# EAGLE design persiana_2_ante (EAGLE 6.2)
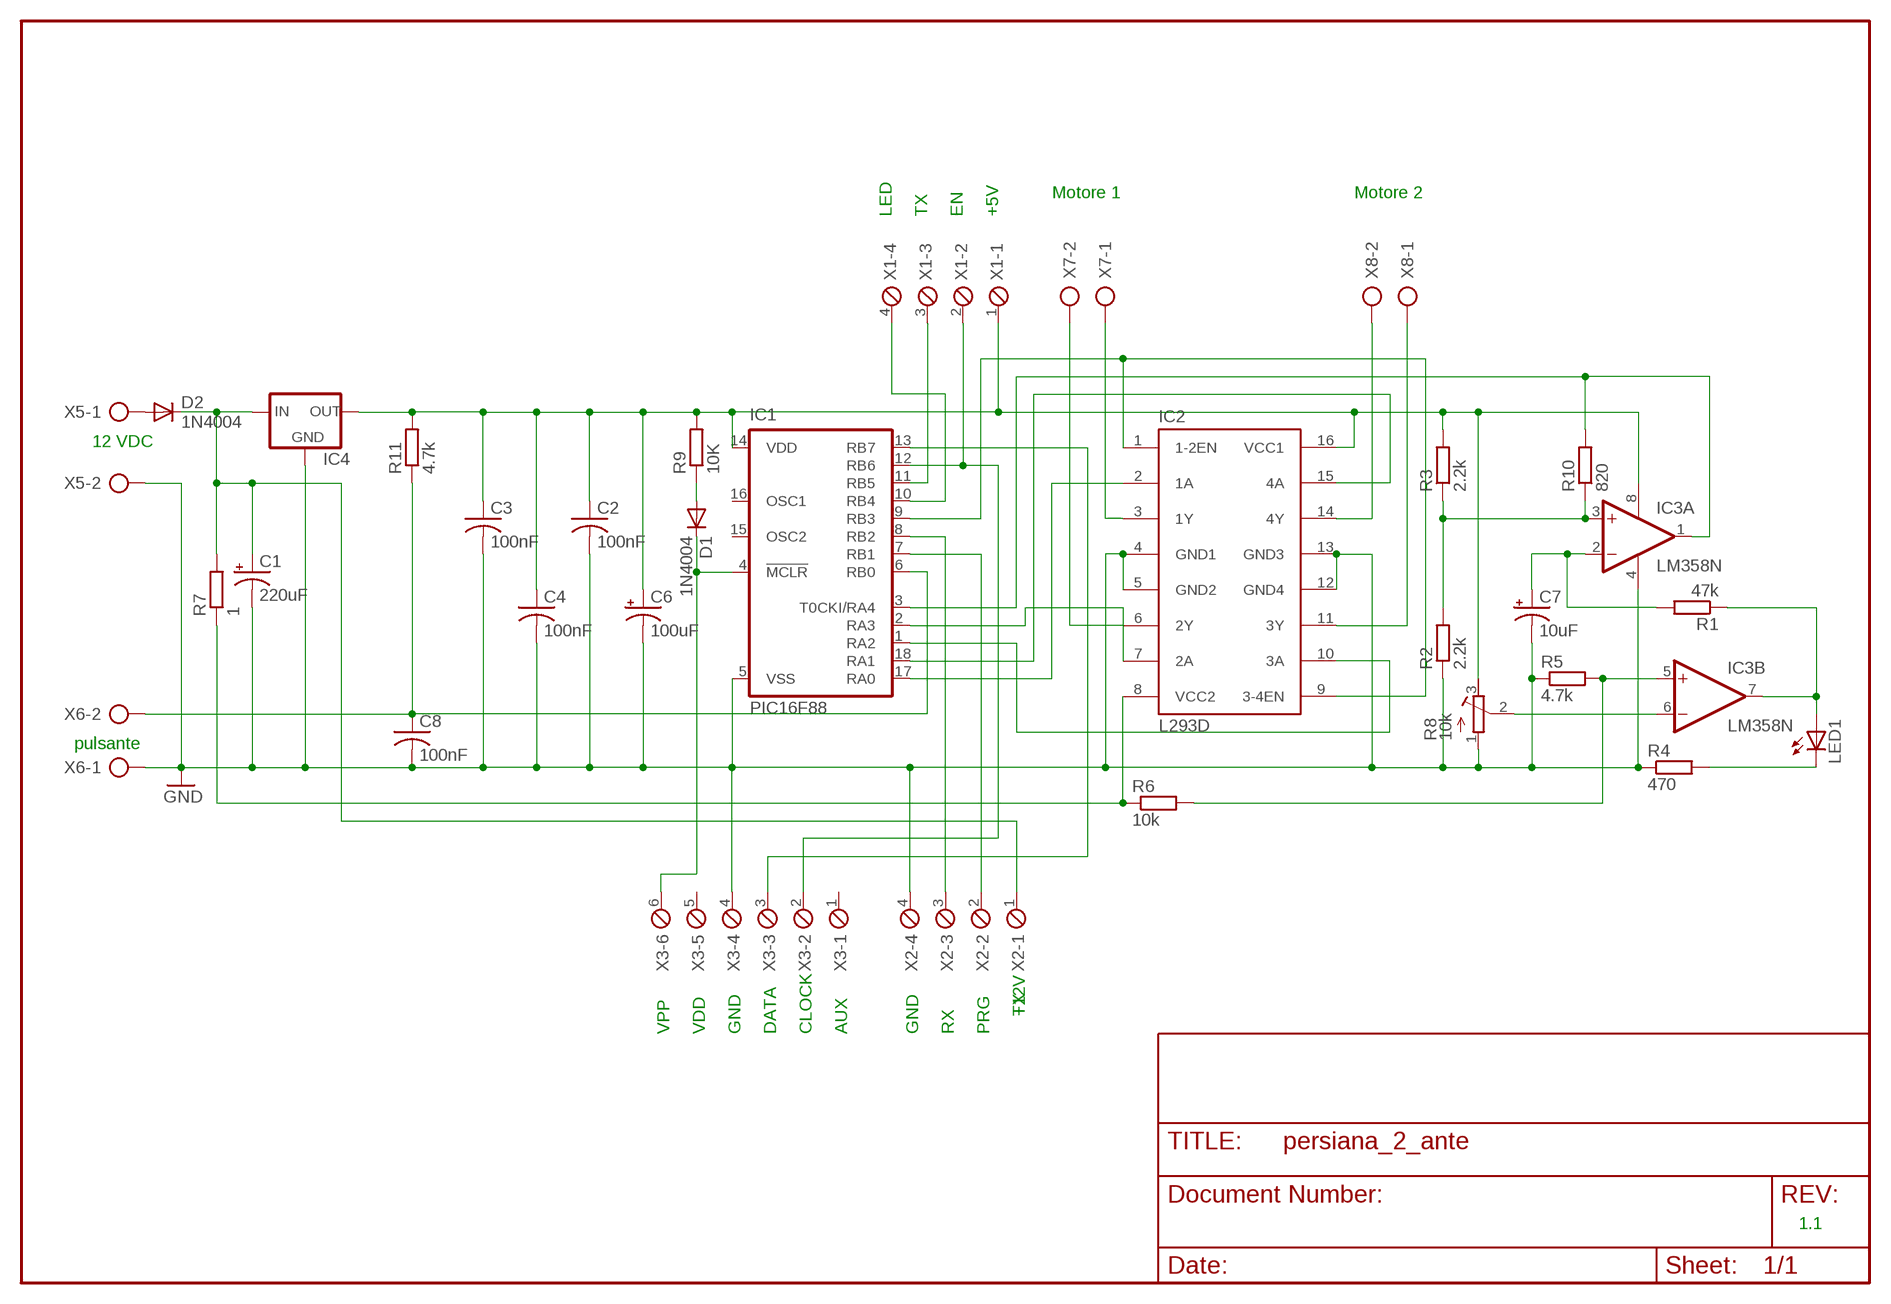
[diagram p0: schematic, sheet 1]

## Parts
C1  220uF  CPOL-USE5-10.5  [E5-10,5]
C2  100nF  C-US050-024X044  [C050-024X044]
C3  100nF  C-US050-024X044  [C050-024X044]
C4  100nF  C-US050-024X044  [C050-024X044]
C6  100uF  CPOL-USE5-10.5  [E5-10,5]
C7  10uF  CPOL-USE5-8.5  [E5-8,5]
C8  100nF  C-US050-024X044  [C050-024X044]
D1  1N4004  [DO41-10]
D2  1N4004  [DO41-10]
IC1  PIC16F88  PIC16F84AP  [DIL18]
IC2  L293D  [DIL16]
IC3  LM358N  [DIL08]
IC4  78XXS  [78XXS]
LED1  LED3MM  [LED3MM]
R1  47k  R-EU_0207/10  [0207/10]
R2  2.2k  R-EU_0207/10  [0207/10]
R3  2.2k  R-EU_0207/10  [0207/10]
R4  470  R-EU_0207/10  [0207/10]
R5  4.7k  R-EU_0207/10  [0207/10]
R6  10k  R-EU_0207/10  [0207/10]
R7  1  R-EU_0411/15  [0411/15]
R8  10k  R-TRIMM3296W  [RTRIM3296W]
R9  10K  R-EU_0207/10  [0207/10]
R10  820  R-EU_0207/10  [0207/10]
R11  4.7k  R-EU_0207/10  [0207/10]
X1  MPT4  [4POL254]
X2  MPT4  [4POL254]
X3  MPT6  [6POL254]
X5  AK500/2  [AK500/2]
X6  AK500/2  [AK500/2]
X7  AK500/2  [AK500/2]
X8  AK500/2  [AK500/2]

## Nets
GND: C1.- C2.2 C3.2 C4.2 C6.- C7.- C8.2 IC1.5(VSS) IC2.4(GND1) IC2.5(GND2) IC2.12(GND4) IC2.13(GND3) IC3.4(P:V-) IC4.GND R2.1 R4.1 R5.1 R8.1(E) X2.4 X3.4 X5.2 X6.1
N$1: C1.+ D2.C IC4.IN R7.2 X2.1
N$2: IC2.3(1Y) X7.1
N$3: IC2.6(2Y) X7.2
N$4: C8.1 IC1.6(RB0) R11.1 X6.2
N$6: D1.C IC1.4(!MCLR) X3.6
N$7: IC2.14(4Y) X8.2
N$8: C2.1 C3.1 C4.1 C6.+ IC1.14(VDD) IC2.16(VCC1) IC3.8(P:V+) IC4.OUT R3.2 R8.3(A) R9.2 R11.2 X1.1
N$9: IC2.8(VCC2) R6.1 R7.1
N$10: IC2.11(3Y) X8.1
N$11: IC1.13(RB7) X3.3
N$12: IC1.17(RA0) IC2.2(1A)
N$13: IC1.18(RA1) IC2.15(4A)
N$14: IC1.1(RA2) IC2.10(3A)
N$15: IC1.2(RA3) IC2.7(2A)
N$16: IC3.5(B:+IN) R5.2 R6.2
N$17: IC3.6(B:-IN) R8.2(S)
N$18: C7.+ IC3.2(A:-IN) R1.2
N$19: IC3.7(B:OUT) LED1.A R1.1
N$20: IC3.3(A:+IN) R2.2 R3.1 R10.1
N$21: IC1.11(RB5) X1.3
N$22: IC1.7(RB1) X2.2
N$23: IC1.3(T0CKI/RA4) IC3.1(A:OUT) R10.2
N$24: IC1.8(RB2) X2.3
N$25: LED1.K(C) R4.2
N$26: IC1.10(RB4) X1.4
N$27: D1.A R9.1
N$28: D2.A X5.1
N$42: IC1.9(RB3) IC2.1(1-2EN) IC2.9(3-4EN)
N$43: IC1.12(RB6) X1.2 X3.2
Unconnected: IC1.15(OSC2) IC1.16(OSC1) X3.1 X3.5

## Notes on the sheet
- Motore 1 | Motore 2
- LED | TX | EN | +5V
- 12 VDC
- pulsante
- +12V | TX
- VPP | VDD | GND | DATA | CLOCK | AUX | GND | RX | PRG
- 1.1

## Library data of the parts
C1 C6 C7 = rcl:CPOL-US: POLARIZED CAPACITOR, American symbol
C2-C4 C8 = rcl:C-US: CAPACITOR, American symbol
D1 D2 = diode:1N4004: DIODE
IC1 = microchip:PIC16F8*: MICROCONTROLLER 8-Bit PIC16F8X Family - CMOS Flash/EEPROM Pin Compatible : PIC16F83, PIC16CR83, PIC16F84A, PIC16CR84 see also PIC16C*
IC2 = st-microelectronics:L293D: PUSH-PULL 4 CHANNEL DRIVER
IC3 = linear:LM358: OP AMP
IC4 = v-reg:78XXS: VOLTAGE REGULATOR
LED1 = led:LED: LED
R1-R7 R9-R11 = rcl:R-EU_: RESISTOR, European symbol
R8 = rcl:R-TRIMM: Trimm resistor
X1 X2 = con-phoenix-254:MPT4: PHOENIX CONNECTOR; OC_FARNELL: unknown; OC_NEWARK: unknown
X3 = con-phoenix-254:MPT6: PHOENIX CONNECTOR; OC_FARNELL: unknown; OC_NEWARK: unknown
X5-X8 = con-ptr500:AK500/2: CONNECTOR; OC_FARNELL: unknown; OC_NEWARK: unknown

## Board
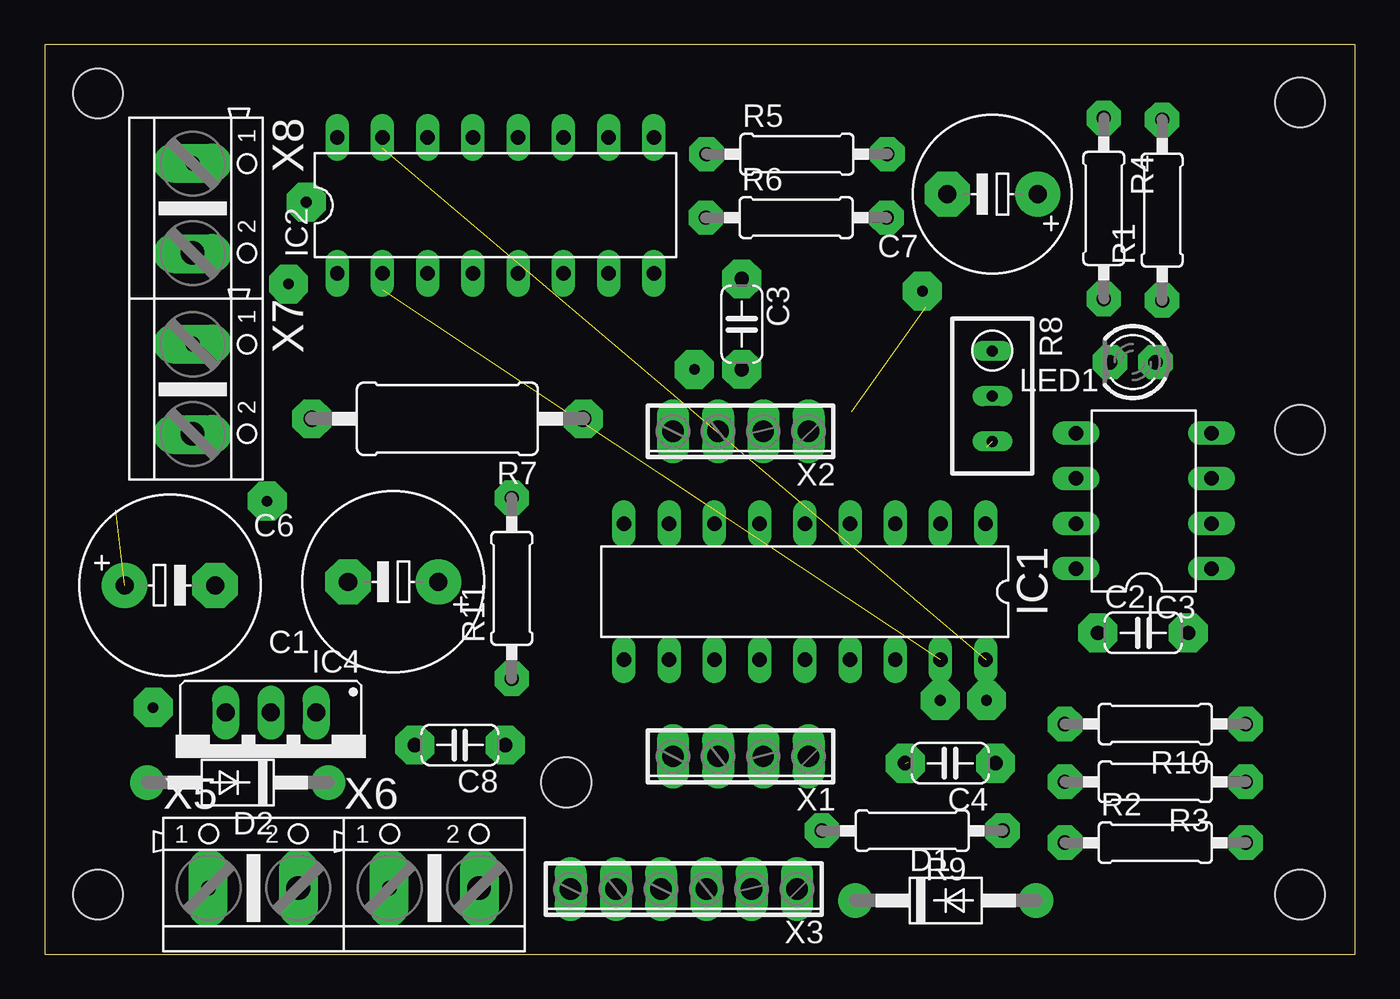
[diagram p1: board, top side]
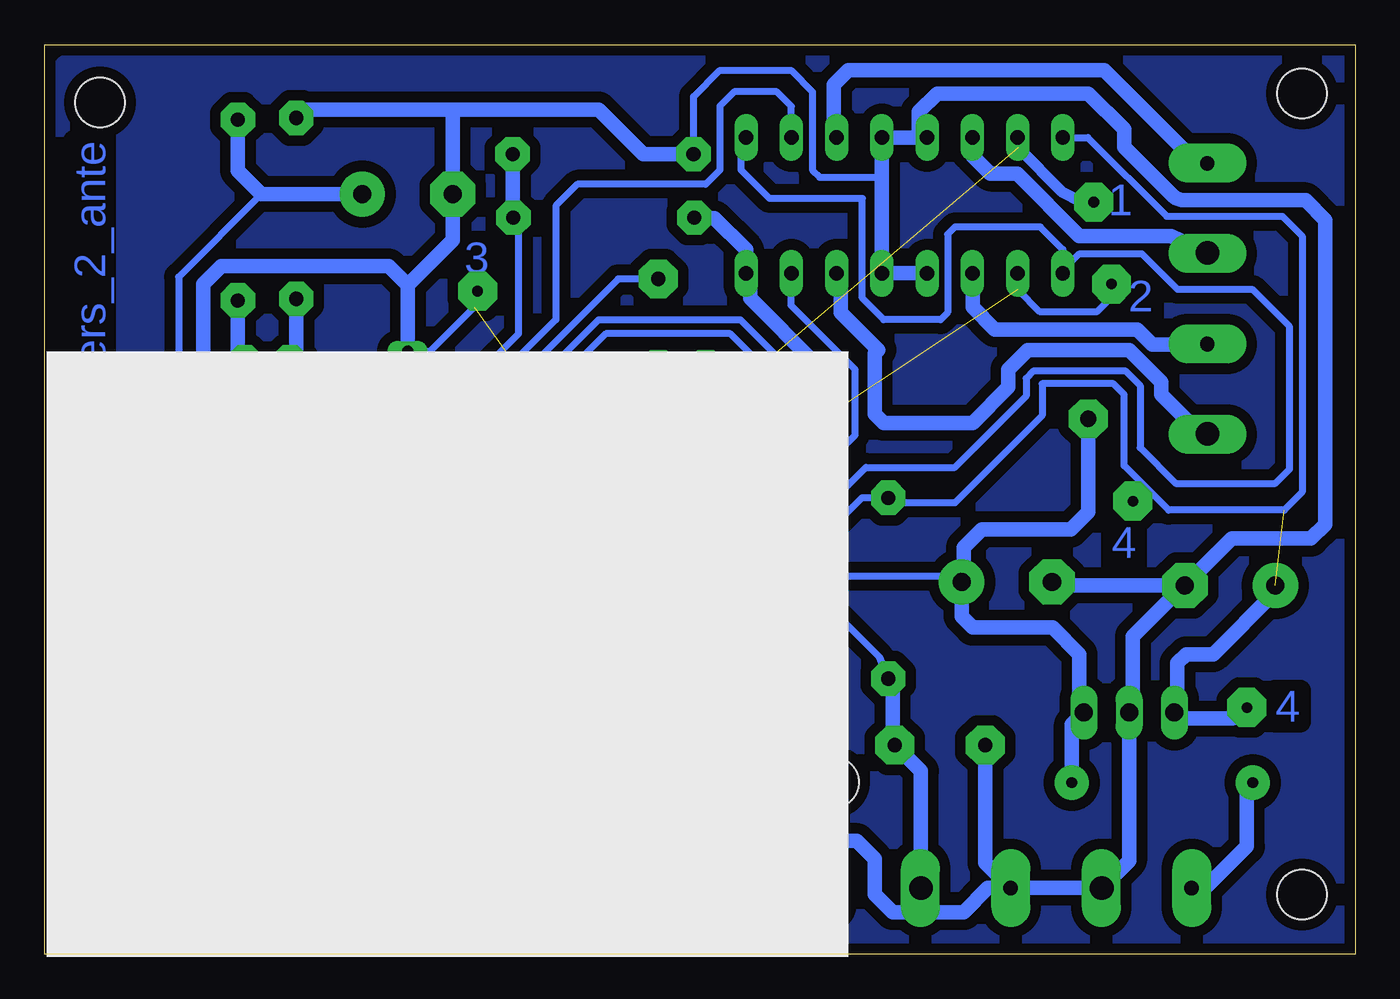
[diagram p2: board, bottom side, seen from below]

Size 73.62 x 51.11 mm. Coordinates in mm from the lower left corner, seen from the top.
Outline: 0,0 73.62,0 73.62,51.11 0,51.11 0,0
Copper layers (1*16): Top 0.035mm / dielectric 1.5mm / Bottom 0.035mm
Design rules: minimum track width 0.6mm, minimum drill 24mil, track to track 8mil, track to pad 8mil, pad to pad 8mil, via to via 8mil, smd to smd 8mil, copper to edge 20mil, drill to drill 8mil, minimum pad ring 10mil, minimum via ring 8mil, stop-mask expansion 4mil, vias tented up to drill 0mil, thermal gap 10mil
Holes 2.8 mm at 3,48.35 70.5,47.85 70.5,3.35 3,3.35 29.3,9.65 70.5,29.45

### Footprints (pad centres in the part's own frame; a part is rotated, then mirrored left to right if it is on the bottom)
E5-10,5 = drill 1.016 pad 2.54: + -2.54,0 | drill 1.016 pad 2.54 octagon: - 2.54,0
C050-024X044 = drill 0.8 pad 2.184 octagon: 1 -2.54,0; 2 2.54,0
E5-8,5 = drill 1.016 pad 2.54: + -2.54,0 | drill 1.016 pad 2.54 octagon: - 2.54,0
DO41-10 = drill 0.6 pad 1.93: A 5.08,0; C -5.08,0
DIL18 = drill 0.813 long: 1 -10.16,-3.81; 2 -7.62,-3.81; 3 -5.08,-3.81; 4 -2.54,-3.81; 5 0,-3.81; 6 2.54,-3.81; 7 5.08,-3.81; 8 7.62,-3.81; 9 10.16,-3.81; 10 10.16,3.81; 11 7.62,3.81; 12 5.08,3.81; 13 2.54,3.81; 14 0,3.81; 15 -2.54,3.81; 16 -5.08,3.81; 17 -7.62,3.81; 18 -10.16,3.81
DIL16 = drill 0.813 long: 1 -8.89,-3.81; 2 -6.35,-3.81; 3 -3.81,-3.81; 4 -1.27,-3.81; 5 1.27,-3.81; 6 3.81,-3.81; 7 6.35,-3.81; 8 8.89,-3.81; 9 8.89,3.81; 10 6.35,3.81; 11 3.81,3.81; 12 1.27,3.81; 13 -1.27,3.81; 14 -3.81,3.81; 15 -6.35,3.81; 16 -8.89,3.81
DIL08 = drill 0.813 long: 1 -3.81,-3.81; 2 -1.27,-3.81; 3 1.27,-3.81; 4 3.81,-3.81; 5 3.81,3.81; 6 1.27,3.81; 7 -1.27,3.81; 8 -3.81,3.81
78XXS = drill 1.016 long: GND 0,-2.54; IN -2.54,-2.54; OUT 2.54,-2.54
LED3MM = drill 0.813 pad 1.93 octagon: A -1.27,0; K 1.27,0
0207/10 = drill 0.8 pad 1.93 octagon: 1 -5.08,0; 2 5.08,0
0411/15 = drill 0.914 pad 2.184 octagon: 1 -7.62,0; 2 7.62,0
RTRIM3296W = drill 0.61 long: 1 0,-2.54; 2 0,0; 3 0,2.54
4POL254 = drill 1.2 long: 1 -3.81,0; 2 -1.27,0; 3 1.27,0; 4 3.81,0 | drill 0.8 pad 1.778 long: P$1 -3.81,0; P$2 -1.27,0; P$3 1.27,0; P$4 3.81,0
6POL254 = drill 1.2 pad 1.778 long: 1 -6.35,0; 2 -3.81,0; 3 -1.27,0; 4 1.27,0; 5 3.81,0; 6 6.35,0
AK500/2 = drill 0.8 pad 1.016 long: 1 -2.515,0 | drill 1.321 long: 2 2.515,0 | drill 0.8 pad 2.184 long: P$2 2.54,0; P$3 -2.54,0

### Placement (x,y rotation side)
C1  19.58,20.91 180 top
C2  61.7,18.05 0 top
C3  39.16,35.4 270 top
C4  50.87,10.73 180 top
C6  7.04,20.72 0 top
C7  53.23,42.7 180 top
C8  23.33,11.74 180 top
D1  50.61,3.01 0 top
D2  10.85,9.64 180 top
IC1  42.7,20.36 180 top
IC2  25.33,42.07 0 top
IC3  61.74,25.46 90 top
IC4  12.71,11.03 180 top
LED1  61.11,33.26 180 top
R1  62.77,41.8 90 top
R2  62.38,6.26 0 top
R3  62.38,9.68 180 top
R4  59.49,41.9 270 top
R5  42.25,44.95 0 top
R6  42.22,41.38 0 top
R7  22.63,30.08 180 top
R8  53.23,31.35 180 top
R9  48.73,6.93 180 top
R10  62.38,12.93 180 top
R11  26.24,20.55 90 top
X1  39.1,11.11 180 top
X2  39.1,29.37 180 top
X3  35.9,3.65 180 top
X5  11.73,3.71 0 top
X6  21.9,3.71 0 top
X7  8.32,31.75 270 top
X8  8.32,41.91 270 top

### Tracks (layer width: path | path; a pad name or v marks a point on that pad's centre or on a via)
GND  (2 unrouted)
  Bottom 0.406: IC3.4 63.72,29.27 62.1,27.65 62.1,23.65 62.9,22.85 67.3,22.85 67.7,22.45 67.7,19.25 66.5,18.05 C2.2 | R5.1 37.17,48.18 35.7,49.65 31.7,49.65 30.5,48.45 30.5,44.05 30.1,43.65 26.6,43.65 | IC1.5 42.7,25.85 45.3,28.45 45.3,30.45 42.89,32.86 C3.2 36.71,32.86 35.3,30.8 X2.4 | R8.1 51.96,33.89 49.5,36.35
  Bottom 0.813: IC2.4 26.09,38.26 26.5,37.85 | IC2.5 26.6,43.65 IC2.12 24.53,45.88 | IC2.5 26.6,37.95 26.5,37.85 | 26.5,37.85 26.5,38.16 IC2.5 | IC2.13 24.53,45.88 | C6.- 6.95,23.35 2.5,23.35 1.7,24.15 1.7,41.25 2.8,42.35 9.59,42.35 arc45 10.29,42.64 13,45.35 13,46.35 15,48.35 23.5,48.35 24.53,47.32 24.53,45.88 | C6.- 16.84,20.72 C1.- | C6.- 9.63,20.72 12.5,17.85 12.5,13.79 IC4.GND 12.71,5.25 X5.2 X6.1 | X3.4 34.5,3.78 34.5,5.85 34,6.35 28,6.35 27,5.35 27,3.35 26,2.35 22,2.35 20.64,3.71 X6.1 | C8.2 20.79,5.12 X6.1 | R5.1 40,44.95 42.5,47.45 50.7,47.45 | 50.7,47.45 59.02,47.45 R4.1 | 50.7,47.45 50.69,47.45 C7.- 50.69,40.12 53.23,37.59 | 53.23,37.59 R8.1 | 48.5,10.8 49.15,10.55 51,8.95 54.61,8.95 R2.1 64.24,13.2 C2.2 | IC3.4 65.55,30.2 64.7,31.05 64.7,37.65 63.7,38.65 54.3,38.65 53.23,37.59
N$1
  Bottom 0.406: 42.91,28.86 X2.1 42.9,27.25 42.1,26.45 39.7,26.45 38.9,25.65 38.9,22.05 38.1,21.25 22.46,21.25 C1.+
  Bottom 0.813: R7.2 15.01,24.84 16,23.85 21,23.85 22,22.85 22,21.04 C1.+ 22.12,18.97 21.5,18.35 17,18.35 15.5,16.85 15.5,13.82 IC4.IN 15.93,12.9 D2.C
N$2
  Bottom 0.813: X7.1 11.41,34.26 12.25,35.1 20.25,35.1 21.5,36.35 21.5,38.24 IC2.3
N$3
  Bottom 0.813: X7.2 8.68,29.23 10.9,31.45 10.9,32.15 12.7,33.95 18.4,33.95 19.5,32.85 19.5,31.85 21.5,29.85 26.5,29.85 27,30.35 27,33.75 26.8,33.95 28.9,36.05 28.9,38.02 IC2.6
N$4
  Bottom 0.406: R11.1 26.72,16.67 30.1,20.05 38.5,20.05 40.5,22.05 40.5,23.83 IC1.6
  Bottom 0.813: X6.2 24.41,10.28 C8.1 25.89,11.74 26,11.85 26,15.23 R11.1
N$5  (via drill 0.6 pad 2.18)
  other vias: 12.5,25.45
N$6
  Bottom 0.406: D1.C 45.53,4.38 46.5,5.35 46.5,11.35 44,13.85 44,20.85 45,21.85 45,23.94 IC1.4
  Bottom 0.813: X3.6 29.55,1.8 30.5,0.85 45,0.85 45.5,1.35 45.5,2.98 D1.C
N$7
  Bottom 0.813: IC2.14 21.52,44.87 20.5,43.85 19,43.85 15.5,40.35 10.36,40.35 X8.2
N$8  (2 unrouted)
  Bottom 0.406: IC2.16 15.03,45.88 10.6,41.45 4.1,41.45 3,40.35 3,25.95 4,24.95 10.5,24.95 13,27.45 13,31.45 13.6,32.05 17.6,32.05 17.6,30.25 22.5,25.35 25.96,25.35 R11.2 27.72,25.63 31.3,22.05 33.3,22.05 33.9,22.25 33.9,27.45 33.3,28.05 33.3,33.05 35.1,34.85 42.1,34.85 47.7,29.25 47.7,26.85 | C2.1 59.16,20.42 IC3.8 | C4.1 53.41,11.54 52.15,12.55 48.55,12.55 46.5,14.85 46.5,26.05 | 46.5,26.05 46.1,26.45 44.9,26.45 44.1,25.65 44.1,22.85 42.9,21.65 42.9,16.76 IC1.14 | 46.5,26.05 47.3,26.85 47.7,26.85 | 47.7,26.85 48.5,26.85 48.9,26.45 48.9,22.85 49.7,22.05 51.3,22.05 51.7,22.45 51.7,27.27 R8.3 | C3.1 41.41,37.94 50.9,28.45 52.88,28.45
  Bottom 0.813: C6.+ 4.5,20.35 8,16.85 9.5,16.85 10,16.35 10,13.75 IC4.OUT | IC1.14 42.7,11.32 X1.1 42.91,7.68 R9.2 | C2.1 59.16,16.19 60.5,14.85 60.5,12.88 R3.2 56.26,10.73 C4.1
N$9
  Bottom 0.813: R7.1 30.25,33.1 34,36.85 34,38.04 IC2.8 34.22,39.57 36,41.35 37.11,41.35 R6.1
N$10
  Bottom 0.813: X8.1 8.87,44.42 14.1,49.65 28.5,49.65 29.3,48.85 29.3,46.04 IC2.11
N$11
  Bottom 0.813: IC1.13 40.16,17.69 39,18.85 31.5,18.85 30.5,17.85 30.5,13.35 33,10.85 33,9.85 34.5,8.35 35.5,8.35 37,6.85 37,3.82 X3.3
N$12  (1 unrouted)
  Bottom 0.406: IC2.2 18.98,37.33 17.75,36.1 14.5,36.1 14,36.6
N$13  (1 unrouted)
  Bottom 0.61: IC2.15 arc-45 18.95,45.8 18.95,45.3 16.5,42.85 15.35,42.25
N$14
  Bottom 0.406: IC2.10 31.68,47.63 32.5,48.45 34.9,48.45 35.7,47.65 35.7,44.05 36.5,43.25 43.7,43.25 44.9,42.05 44.9,35.65 50.5,30.05 54.1,30.05 54.9,29.25 54.9,26.22 IC1.1
N$15
  Bottom 0.406: IC2.7 31.7,38.24 31.7,36.45 28.1,32.85 28.1,29.15 29.3,27.95 30.9,27.95 32.1,29.15 32.1,33.2 34.55,35.65 42.5,35.65 50.5,27.65 50.5,26.82 50.32,26.63 IC1.2
N$16
  Bottom 0.406: IC3.5 57.93,30.42 55.5,32.85 49,32.85 47,34.85 47,41.08 R6.2
  Bottom 0.813: R5.2 47.33,41.41 R6.2
N$17
  Bottom 0.406: 53.6,31.35 R8.2 53.33,31.25 54.9,31.25 55.7,30.45 55.7,27.65 56.5,26.85 57.81,26.85 IC3.6
N$18
  Bottom 0.406: IC3.2 65.41,24.05 63.7,24.05 62.9,24.85 62.9,26.85 64.1,28.05 66.9,28.05 67.5,28.65 67.5,30.35 66.1,31.75 66.1,38.05 61.45,42.7
  Bottom 0.813: R1.2 62.77,44.02 61.45,42.7 C7.+
N$19
  Bottom 0.813: R1.1 62.77,33.65 LED1.A 62.39,29.73 61.1,28.45 61.1,28.25 60.9,28.05 | 60.9,28.05 60.9,28.25 | 60.9,28.05 60.9,25.05 60.1,24.25 57.98,24.25 IC3.7
N$20
  Bottom 0.813: R2.2 R3.1 R10.1 | 67.5,12.96 R10.1 | IC3.3 67.42,26.73 68.7,25.45 68.7,14.16 R10.1
N$21
  Bottom 0.813: IC1.11 35.08,15.27 38,12.35 38,11.28 X1.3
N$22
  Bottom 0.813: IC1.7 37.62,25.77 40.5,28.65 40.5,29.23 X2.2
N$23
  Bottom 0.406: 52.6,19.75 55,17.35 55,15.23 R10.2 | IC3.1 61.7,21.65 60.5,22.85 55.7,22.85 52.6,19.75 | IC1.3 47.78,21.97 48.9,20.85 51.5,20.85 52.6,19.75
N$24
  Bottom 0.813: IC1.8 35.08,25.43 37.7,28.05 37.7,29.24 X2.3
N$25
  Bottom 0.813: R4.2 59.49,33.62 LED1.K
N$26
  Bottom 0.813: IC1.10 32.54,13.86 X1.4
N$27
  Bottom 0.813: R9.1 53.81,4.89 D1.A
N$28
  Bottom 0.813: X5.1 8.44,3.71 6.1,6.05 6.1,9.31 D2.A
N$29  (via drill 0.6 pad 2.18)
  other vias: 6.1,13.85
N$30
  Bottom 0.813: 9.9,13.25 6.9,13.25 6.5,13.65
N$42
  Bottom 0.406: 34.1,44.85 34.1,45.76 IC2.9 34.5,45.6 34.5,44.05 32.9,42.45 27.7,42.45 27.7,36.85 26.5,35.65 23.3,35.65 22.9,36.05 22.9,40.45 22.5,40.85 17.7,40.85 16.44,39.59 IC2.1 16.44,38.41 15.5,39.35 12,39.35 10,37.35 5.8,37.35 3.7,35.25 3.7,27.25 4.5,26.45 10.1,26.45 12.1,28.45 12.1,31.95 12.9,32.75 18.1,32.75 18.5,32.35 18.5,31.35 22.5,27.35 27.5,27.35 30.68,24.17 IC1.9
N$43
  Bottom 0.813: IC1.12 37.62,15.73 40,13.35 40,11.48 X1.2 40.5,10.98 40.5,8.85 39.71,8.06 X3.2
S$1
  pour Bottom (isolate 0.61): 1,50.35 72,50.35 arc-90 73,49.35 73,0.35 1.5,0.35 arc-90 0.5,1.35 0.5,50.35
S$2  (via drill 0.6 pad 2.18)
  other vias: 14.7,42.25
S$3  (via drill 0.6 pad 2.18)
  other vias: 13.7,37.65
S$4  (via drill 0.6 pad 2.18)
  other vias: 50.3,14.25
S$5  (via drill 0.6 pad 2.18)
  other vias: 52.9,14.25
S$6  (via drill 0.6 pad 2.18)
  other vias: 49.3,37.25
S$7  (via drill 0.6 pad 2.18)
  other vias: 36.5,32.85

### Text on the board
Bottom: pers_2_ante | 1 | 3 | 2 | 3 | 4 | 2 | 1 | 4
